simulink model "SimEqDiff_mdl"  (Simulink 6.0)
settings: Solver=ode45  StartTime=0.0  StopTime=10.0  MaxStep=1e-2  RelTol=1e-3
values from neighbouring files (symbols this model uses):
  ddy0 = 0    [SimEqDiff.m]
  dy0 = 3    [SimEqDiff.m]
  y0 = -2    [SimEqDiff.m]

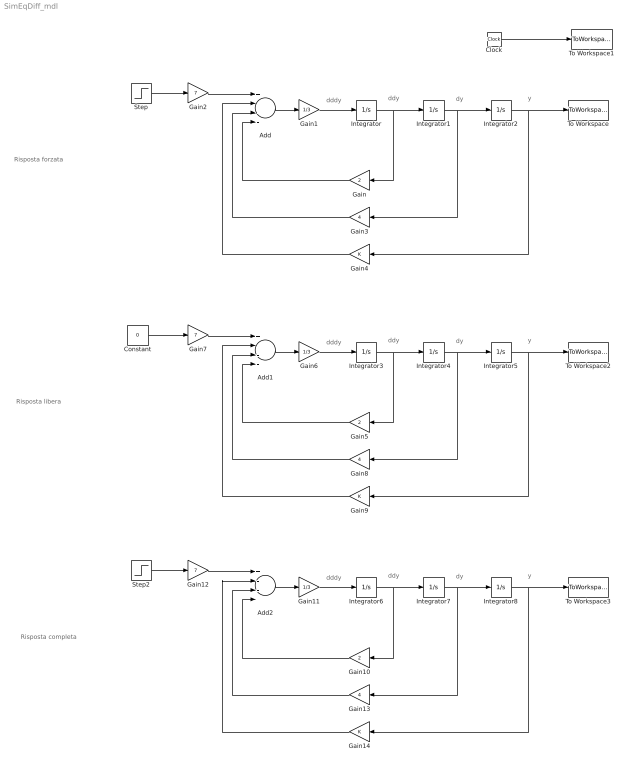
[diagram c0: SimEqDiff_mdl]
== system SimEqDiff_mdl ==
  note: dddy
  note: ddy
  note: dy
  note: y
  note: Risposta forzata
  note: dddy
  note: ddy
  note: dy
  note: y
  note: Risposta libera
  note: dddy
  note: ddy
  note: dy
  note: y
  note: Risposta completa
  Add : Sum  Inputs=+---  OutDataType=sfix(16)  OutScaling=2^-10
  Add1 : Sum  Inputs=+---  OutDataType=sfix(16)  OutScaling=2^-10
  Add2 : Sum  Inputs=+---  OutDataType=sfix(16)  OutScaling=2^-10
  Clock : Clock
  Constant : Constant  Value=0  OutDataType=sfix(16)  OutScaling=2^0
  Gain : Gain  Orientation=left  Gain=2  ParameterDataType=sfix(16)  ParameterScaling=2^0  OutDataType=sfix(16)  OutScaling=2^0
  Gain1 : Gain  Gain=1/3  ParameterDataType=sfix(16)  ParameterScaling=2^0  OutDataType=sfix(16)  OutScaling=2^0
  Gain10 : Gain  Orientation=left  Gain=2  ParameterDataType=sfix(16)  ParameterScaling=2^0  OutDataType=sfix(16)  OutScaling=2^0
  Gain11 : Gain  Gain=1/3  ParameterDataType=sfix(16)  ParameterScaling=2^0  OutDataType=sfix(16)  OutScaling=2^0
  Gain12 : Gain  Gain=7  ParameterDataType=sfix(16)  ParameterScaling=2^0  OutDataType=sfix(16)  OutScaling=2^0
  Gain13 : Gain  Orientation=left  Gain=4  ParameterDataType=sfix(16)  ParameterScaling=2^0  OutDataType=sfix(16)  OutScaling=2^0
  Gain14 : Gain  Orientation=left  ParameterDataType=sfix(16)  ParameterScaling=2^0  OutDataType=sfix(16)  OutScaling=2^0
  Gain2 : Gain  Gain=7  ParameterDataType=sfix(16)  ParameterScaling=2^0  OutDataType=sfix(16)  OutScaling=2^0
  Gain3 : Gain  Orientation=left  Gain=4  ParameterDataType=sfix(16)  ParameterScaling=2^0  OutDataType=sfix(16)  OutScaling=2^0
  Gain4 : Gain  Orientation=left  ParameterDataType=sfix(16)  ParameterScaling=2^0  OutDataType=sfix(16)  OutScaling=2^0
  Gain5 : Gain  Orientation=left  Gain=2  ParameterDataType=sfix(16)  ParameterScaling=2^0  OutDataType=sfix(16)  OutScaling=2^0
  Gain6 : Gain  Gain=1/3  ParameterDataType=sfix(16)  ParameterScaling=2^0  OutDataType=sfix(16)  OutScaling=2^0
  Gain7 : Gain  Gain=7  ParameterDataType=sfix(16)  ParameterScaling=2^0  OutDataType=sfix(16)  OutScaling=2^0
  Gain8 : Gain  Orientation=left  Gain=4  ParameterDataType=sfix(16)  ParameterScaling=2^0  OutDataType=sfix(16)  OutScaling=2^0
  Gain9 : Gain  Orientation=left  ParameterDataType=sfix(16)  ParameterScaling=2^0  OutDataType=sfix(16)  OutScaling=2^0
  Integrator : Integrator
  Integrator1 : Integrator
  Integrator2 : Integrator
  Integrator3 : Integrator  InitialCondition=ddy0
  Integrator4 : Integrator  InitialCondition=dy0
  Integrator5 : Integrator  InitialCondition=y0
  Integrator6 : Integrator  InitialCondition=ddy0
  Integrator7 : Integrator  InitialCondition=dy0
  Integrator8 : Integrator  InitialCondition=y0
  Step : Step  SampleTime=0
  Step2 : Step  SampleTime=0
  To Workspace : ToWorkspace  VariableName=yf  SampleTime=-1  SaveFormat=Array
  To Workspace1 : ToWorkspace  VariableName=time  SampleTime=-1  SaveFormat=Array
  To Workspace2 : ToWorkspace  VariableName=yl  SampleTime=-1  SaveFormat=Array
  To Workspace3 : ToWorkspace  VariableName=yc  SampleTime=-1  SaveFormat=Array
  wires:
  Integrator/1 -> Integrator1/1, Gain/1
  Integrator1/1 -> Integrator2/1, Gain3/1
  Gain1/1 -> Integrator/1
  Add/1 -> Gain1/1
  Gain/1 -> Add/4
  Gain3/1 -> Add/3
  Integrator2/1 -> Gain4/1, To Workspace/1
  Gain4/1 -> Add/2
  Clock/1 -> To Workspace1/1
  Gain2/1 -> Add/1
  Step/1 -> Gain2/1
  Integrator3/1 -> Integrator4/1, Gain5/1
  Integrator4/1 -> Integrator5/1, Gain8/1
  Gain6/1 -> Integrator3/1
  Add1/1 -> Gain6/1
  Gain5/1 -> Add1/4
  Gain8/1 -> Add1/3
  Integrator5/1 -> Gain9/1, To Workspace2/1
  Gain9/1 -> Add1/2
  Gain7/1 -> Add1/1
  Constant/1 -> Gain7/1
  Integrator6/1 -> Integrator7/1, Gain10/1
  Integrator7/1 -> Integrator8/1, Gain13/1
  Gain11/1 -> Integrator6/1
  Add2/1 -> Gain11/1
  Gain10/1 -> Add2/4
  Gain13/1 -> Add2/3
  Integrator8/1 -> Gain14/1, To Workspace3/1
  Gain14/1 -> Add2/2
  Gain12/1 -> Add2/1
  Step2/1 -> Gain12/1
